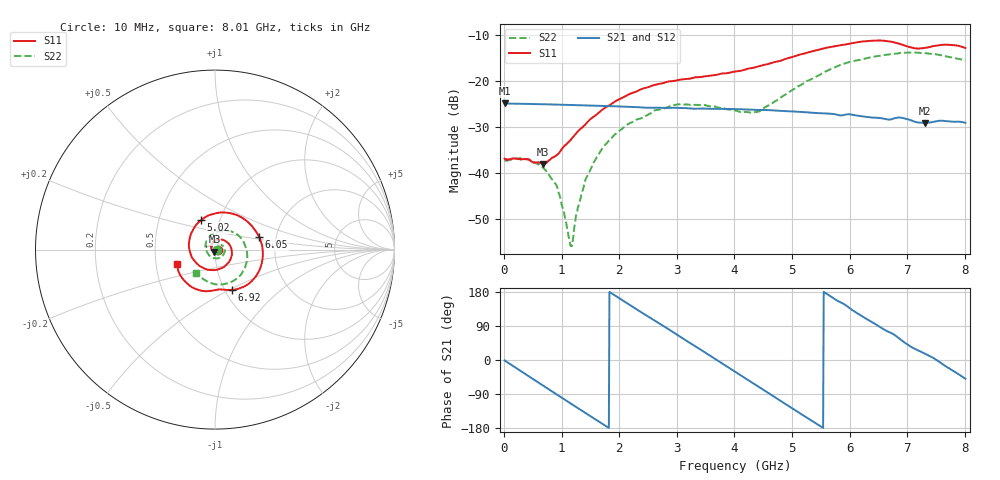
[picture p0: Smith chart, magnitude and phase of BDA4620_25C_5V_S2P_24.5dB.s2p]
!Agilent Technologies,E5071B,MY42404982,A.09.10
!Date: Wed May 06 09:03:43 2026
!Data & Calibration Information:
!Freq	S11:SOLT2(ON)	S21:SOLT2(ON)	S12:SOLT2(ON)	S22:SOLT2(ON)
# Hz S RI R 50
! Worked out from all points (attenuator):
!   801 points, 10 MHz to 8.01 GHz, reference 50 ohm
!   highest |S21| = -24.89 dB at 10 MHz (marker M1); lowest = -29.1 dB at 7.31 GHz (marker M2)
!   lowest |S11| = -38.1 dB at 680 MHz (marker M3), VSWR 1.03, Z = 49.7 - j1.2 ohm
!   |S11| at or under -10 dB: start of sweep to end of sweep
!   |S22| runs from -55.8 to -13.9 dB; largest |S21 - S12| = 0.00028
!   S11 on the Smith chart (normalised r, x): 10 MHz: 1.03, -0.00; 5.02 GHz: 0.81, +0.28; 6.05 GHz: 1.63, +0.25; 6.92 GHz: 1.08, -0.52; 8.01 GHz: 0.64, -0.11
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1e7  0.0144 -0.000976  0.0569 -0.0012  0.057 -0.00122  0.0135 -0.000468
4.3e8  0.0078 -0.0117  0.0411 -0.0383  0.0411 -0.0384  0.0132 -0.00481
6.8e8  -0.00295 -0.0121  0.0211 -0.0515  0.0211 -0.0516  0.0092 -0.00663
9.3e8  -0.0149 -0.00547  -0.00225 -0.0552  -0.00237 -0.0553  0.00348 -0.00589
1.16e9  -0.0215 0.00827  -0.0231 -0.0496  -0.0232 -0.0496  -0.00139 -0.000835
1.35e9  -0.0214 0.0225  -0.0375 -0.0393  -0.0375 -0.0393  -0.00337 0.00494
1.53e9  -0.0151 0.0368  -0.0471 -0.026  -0.0472 -0.026  -0.00314 0.0115
1.77e9  0.00256 0.0516  -0.053 -0.0051  -0.0531 -0.00508  0.000998 0.0206
2.15e9  0.0449 0.0541  -0.0446 0.0273  -0.0447 0.0274  0.0174 0.0293
2.68e9  0.0921 0.00224  -0.00701 0.0506  -0.00699 0.0506  0.0445 0.0192
3.07e9  0.0828 -0.0615  0.0251 0.0441  0.0253 0.0441  0.0555 -0.00675
4.01e9  -0.0894 -0.0882  0.0424 -0.0252  0.0424 -0.0253  -0.0108 -0.0466
4.42e9  -0.1434 0.00379  0.0161 -0.0456  0.0161 -0.0456  -0.0448 -0.0126
5.02e9  -0.0772 0.1648  -0.0293 -0.0361  -0.0294 -0.0362  -0.0293 0.0752
5.35e9  0.0288 0.2064  -0.0427 -0.0146  -0.0427 -0.0146  0.0232 0.1026
6.05e9  0.2457 0.0714  -0.0284 0.0321  -0.0285 0.0321  0.154 0.0519
6.37e9  0.2624 -0.0678  -0.00804 0.0393  -0.00806 0.0393  0.1784 -0.016
6.68e9  0.1877 -0.1901  0.0105 0.0366  0.0105 0.0366  0.1701 -0.0902
6.92e9  0.0957 -0.2252  0.0255 0.0303  0.0256 0.0304  0.141 -0.143
7.31e9  -0.00437 -0.2265  0.0336 0.00991  0.0337 0.00989  0.0508 -0.1921
7.64e9  -0.122 -0.2128  0.0357 -0.00865  0.0358 -0.00873  -0.031 -0.1838
8.01e9  -0.211 -0.0819  0.0228 -0.0266  0.023 -0.0268  -0.1036 -0.1286
